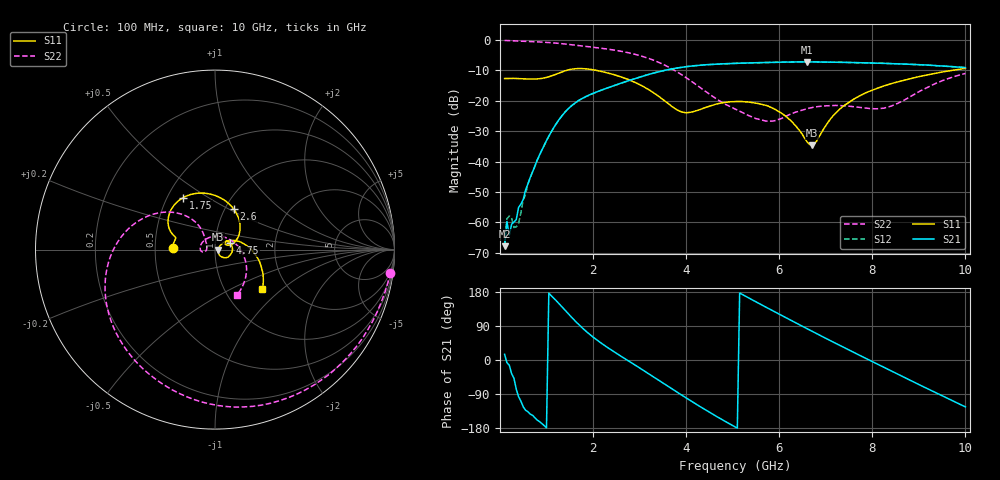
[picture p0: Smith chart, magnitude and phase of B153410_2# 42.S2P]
!  2-Port S-parameters saved by WinCal
! VAR MeasName=S-Parameters (CALIBRATED_DATA) read from VNA (N5245A)
! VAR MeasDate=2016-12-23 10:01:32
! VAR NAME=B153410_2# 42
! VAR FILENAME=B153410_2# 42.S2P
! VAR DATE=2016-12-23 10:01:32
! VAR PHYS_PORTS=1,2
# Hz S DB R 50
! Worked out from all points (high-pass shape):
!   199 points, 100 MHz to 10 GHz, reference 50 ohm
!   highest |S21| = -7.19 dB at 6.6 GHz (marker M1); lowest = -67.9 dB at 100 MHz (marker M2)
!   |S21| within 3 dB of the highest: 3.479 GHz to end of sweep
!   lowest |S11| = -34.6 dB at 6.7 GHz (marker M3), VSWR 1.04, Z = 51.9 - j0.126 ohm
!   |S11| at or under -10 dB: start of sweep to 1.427 GHz; 2.077 GHz to 9.704 GHz (7.627 GHz wide, 129 % of centre)
!   |S22| runs from -26.7 to -0.1 dB; largest |S21 - S12| = 0.0036
!   S11 on the Smith chart (normalised r, x): 100 MHz: 0.62, +0.01; 1.75 GHz: 0.60, +0.39; 2.6 GHz: 1.10, +0.53; 4.75 GHz: 1.18, +0.08; 10 GHz: 1.50, -0.74
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1e8  -12.67 178.1  -67.86 14.8  -67.23 83.6  -0.13 -7.4
1.5e8  -12.65 176.7  -59.77 -7.1  -58.85 22.8  -0.17 -10.9
2e8  -12.63 175.4  -64.28 -13.5  -57.93 14.5  -0.21 -14.3
3e8  -12.62 172.4  -59.92 -48.0  -61.73 -53.5  -0.28 -21.0
3.5e8  -12.65 171.0  -59.13 -76.8  -61.50 -46.0  -0.31 -24.3
4e8  -12.70 170.0  -55.11 -96.7  -60.39 -79.3  -0.34 -27.7
6e8  -12.84 165.7  -47.43 -136.4  -47.37 -139.1  -0.46 -40.8
1e9  -12.30 161.2  -33.08 -178.8  -33.15 -178.6  -0.77 -66.8
1.35e9  -10.38 149.8  -24.60 138.0  -24.58 138.1  -1.22 -89.0
1.75e9  -9.38 121.6  -19.39 86.9  -19.39 86.7  -1.93 -112.3
2.6e9  -12.12 64.8  -14.20 10.0  -14.23 10.1  -3.69 -159.5
3.4e9  -18.39 21.6  -10.48 -52.4  -10.48 -52.3  -7.27 155.9
4e9  -23.94 29.4  -8.77 -100.0  -8.77 -100.0  -12.39 130.0
4.75e9  -20.75 22.8  -7.86 -155.8  -7.86 -155.6  -20.32 128.2
5.05e9  -20.26 7.4  -7.67 -176.6  -7.69 -176.4  -22.70 136.1
5.9e9  -22.74 -38.5  -7.33 127.6  -7.32 127.7  -26.59 -179.9
6.6e9  -33.53 -29.5  -7.19 82.6  -7.21 82.6  -22.60 -170.8
6.7e9  -34.61 -3.7  -7.20 76.2  -7.21 76.2  -22.25 -173.1
7.35e9  -22.10 36.9  -7.34 35.6  -7.34 35.7  -21.62 161.4
8.35e9  -14.62 4.8  -7.74 -25.5  -7.73 -25.2  -22.02 69.2
9.2e9  -11.43 -18.5  -8.25 -76.7  -8.27 -76.5  -15.48 -14.5
1e10  -9.31 -39.4  -9.08 -123.8  -9.08 -123.2  -11.00 -64.5
